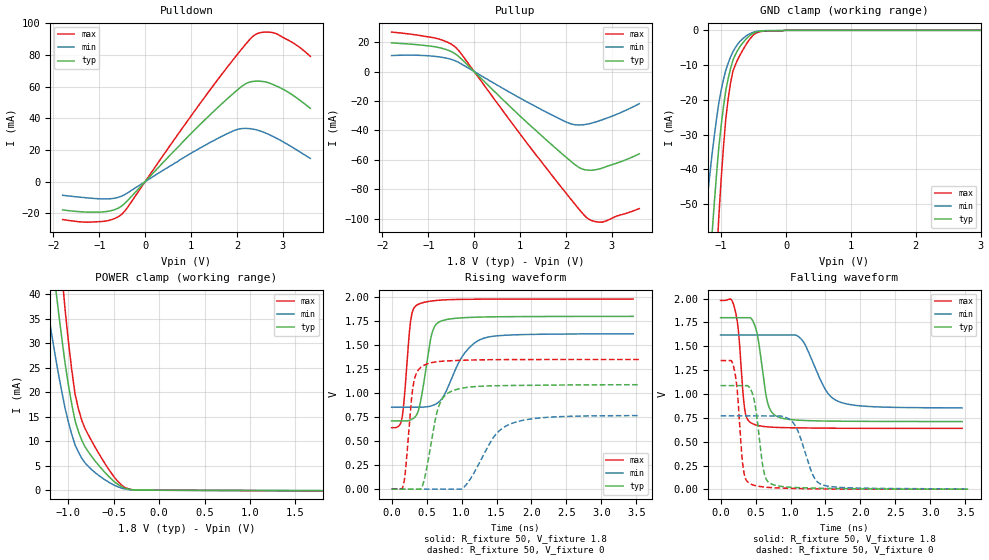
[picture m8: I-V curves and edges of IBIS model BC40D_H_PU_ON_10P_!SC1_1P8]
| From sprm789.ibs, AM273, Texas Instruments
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|   Model Cell BC40D_H_PU_ON_10P_!SC1_1P8
|BC40D_H_PU_ON_10P_!SC1_1P8
[Model]   BC40D_H_PU_ON_10P_!SC1_1P8
Model_type   I/O
Polarity   Non-Inverting
Enable   Active-Low
Vinl =  0.63
Vinh =  1.17
Cref =  15pF
Rref =  100.0000M
Vref =  0V
Vmeas =  0.9
C_comp   2.389419p   2.292106p   2.408415p
|[Input load] weak_pu_on
|[Output drive] fast
|[supplytol] 10
|[temp] ind
[Model Spec]
Vinl   0.63   0.567   0.693
Vinh   1.17   1.053   1.287
[Temperature Range]   25   125   -40
[Voltage Range]   1.8   1.62   1.98
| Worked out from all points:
|   slope of the pulldown table from 0 to 0.27 V, typ, clamps not added: 32.2 ohm
|   slope of the pullup table from 0 to 0.27 V, typ, clamps not added: 32.5 ohm
|   GND clamp passes 1 mA (typ) near -0.52 V on its own axis
|   POWER clamp passes 1 mA (typ) near -0.44 V on its own axis
|   rising waveform, R_fixture 50, V_fixture 1.8: 20-80 % time 145ps typ, 330ps min, 88.9ps max; typ from 0.711 V to 1.8 V
|   rising waveform, R_fixture 50, V_fixture 0: 20-80 % time 176ps typ, 382ps min, 100ps max; typ from 0 V to 1.09 V
|   falling waveform, R_fixture 50, V_fixture 1.8: 20-80 % time 130ps typ, 293ps min, 86ps max; typ from 1.8 V to 0.711 V
|   falling waveform, R_fixture 50, V_fixture 0: 20-80 % time 113ps typ, 213ps min, 82.9ps max; typ from 1.09 V to 0.002 V
| Nom Voltages:
|   VDD=1.1001, VDDS=1.8, VDDS18=1.8, ESD_BIASFET=0, VSS=0, VSSS=0
| Min Voltages:
|   VDD=0.99, VDDS=1.62, VDDS18=1.62, ESD_BIASFET=0, VSS=0, VSSS=0
| Max Voltages:
|   VDD=1.21, VDDS=1.98, VDDS18=1.98, ESD_BIASFET=0, VSS=0, VSSS=0
[POWER_clamp]
|   voltage   I(typ)   I(min)   I(max)
-1.8V     158.8mA    112.5mA    219.8mA
-1.255V   59.97mA    40.01mA    84.9mA
-1.145V   41.92mA    27.42mA    59.75mA
-1.109V   36.32mA    23.63mA    51.82mA
-1.073V   30.96mA    20.05mA    44.15mA
-1.036V   25.83mA    16.67mA    36.75mA
-963.6mV  17.54mA    11.39mA    24.55mA
-890.9mV  12.01mA    7.801mA    16.66mA
-818.2mV  8.875mA    5.6mA      12.63mA
-563.6mV  2.954mA    1.727mA    4.458mA
-272.7mV  55.97uA    39.41uA    57.82uA
1.8V      -99.94uA   -59.68uA   -146.8uA
[Pulldown]
|   voltage   I(typ)   I(min)   I(max)
-1.8V     -17.92mA   -8.674mA   -24.03mA
-927.3mV  -19.22mA   -10.99mA   -25.21mA
-654.5mV  -17.65mA   -10.46mA   -23.22mA
-490.9mV  -14.97mA   -8.904mA   -20.12mA
818.2mV   25.05mA    14.78mA    34.16mA
1.691V    49.7mA     28.87mA    68.59mA
2.127V    60.63mA    33.53mA    84.59mA
2.4V      63.43mA    32.84mA    92.9mA
2.618V    62.99mA    30.74mA    94.47mA
2.836V    60.69mA    27.76mA    93.76mA
3.273V    53.49mA    20.53mA    86.73mA
3.6V      46.26mA    14.64mA    79.11mA
[Pullup]
|   voltage   I(typ)   I(min)   I(max)
-1.8V     19.47mA    10.86mA    26.81mA
-818.2mV  16.61mA    10.18mA    22.5mA
-545.5mV  14.21mA    8.665mA    19.39mA
-381.8mV  11.35mA    6.855mA    15.77mA
1.036V    -31.31mA   -18.66mA   -43.94mA
1.909V    -55.72mA   -32.86mA   -78.99mA
2.182V    -62.87mA   -36.1mA    -89.59mA
2.345V    -66.12mA   -36.26mA   -95.76mA
2.455V    -66.95mA   -35.82mA   -99.33mA
2.618V    -66.9mA    -34.58mA   -101.8mA
2.782V    -65.73mA   -32.89mA   -102.4mA
3.6V      -55.92mA   -21.86mA   -93.15mA
[GND_clamp]
|   voltage   I(typ)   I(min)   I(max)
-1.8V     -270.2mA   -170.2mA   -430.1mA
-1.255V   -91.68mA   -55.92mA   -148.5mA
-1.145V   -59.94mA   -36.46mA   -97.15mA
-1.109V   -50.51mA   -30.84mA   -81.62mA
-1.073V   -41.77mA   -25.67mA   -67.14mA
-1.036V   -33.71mA   -20.94mA   -53.69mA
-927.3mV  -17.15mA   -11.38mA   -25.2mA
-854.5mV  -10.96mA   -7.657mA   -15.09mA
-781.8mV  -7.031mA   -4.995mA   -9.958mA
-563.6mV  -1.569mA   -1.036mA   -2.651mA
-18.18mV  0A         0A         0A
3.6V      0A         0A         0A
[Ramp]
| variable   typ   min   max
dV/dt_f 0.66463363/0.13264571n 0.47012824/0.29953481n 0.81358705/87.601634p
dV/dt_r 0.66384837/0.1782439n 0.48059819/0.39802224n 0.81799537/0.10135541n
R_load = 50
[Rising Waveform]
R_fixture = 50
V_fixture = 1.8
V_fixture_min = 1.62
V_fixture_max = 1.98
|   time   V(typ)   V(min)   V(max)
0s        710.5mV    852.8mV    640.5mV
143.5ps   710.5mV    852.8mV    721.7mV
179.2ps   710.5mV    852.8mV    931.5mV
273.6ps   722.6mV    852.8mV    1.76V
373.4ps   799.3mV    852.8mV    1.923V
571.2ps   1.607V     868.2mV    1.96V
697.6ps   1.748V     923.5mV    1.969V
1.016ns   1.785V     1.389V     1.977V
1.312ns   1.793V     1.571V     1.979V
3.453ns   1.8V       1.618V     1.98V
[Rising Waveform]
R_fixture = 50
V_fixture = 0
V_fixture_min = 0
V_fixture_max = 0
|   time   V(typ)   V(min)   V(max)
0s        0V         0V         3.403mV
168.2ps   0V         0V         41.85mV
312.5ps   0V         0V         1.097V
465.8ps   95.89mV    0V         1.292V
662.5ps   837mV      0V         1.328V
859.1ps   1.021V     0V         1.338V
1.051ns   1.057V     33.52mV    1.343V
1.47ns    1.077V     552.6mV    1.349V
1.714ns   1.08V      683.4mV    1.35V
3.542ns   1.088V     766.1mV    1.351V
[Falling Waveform]
R_fixture = 50
V_fixture = 1.8
V_fixture_min = 1.62
V_fixture_max = 1.98
|   time   V(typ)   V(min)   V(max)
0s        1.8V       1.619V     1.981V
202.5ps   1.8V       1.619V     1.896V
255.7ps   1.8V       1.619V     1.659V
347ps     1.8V       1.619V     831.8mV
449.6ps   1.781V     1.619V     691.7mV
673.3ps   907.3mV    1.619V     655.6mV
807.1ps   765.1mV    1.619V     649.8mV
1.149ns   724.1mV    1.58V      645mV
1.693ns   715.1mV    919.7mV    641.1mV
3.453ns   711.3mV    854.8mV    639.8mV
[Falling Waveform]
R_fixture = 50
V_fixture = 0
V_fixture_min = 0
V_fixture_max = 0
|   time   V(typ)   V(min)   V(max)
0s        1.089V     770.9mV    1.351V
189.1ps   1.089V     770.9mV    1.278V
238.1ps   1.089V     770.9mV    1.041V
324.3ps   1.089V     770.9mV    219.8mV
426.3ps   1.055V     770.9mV    58.32mV
620.7ps   180.8mV    770.9mV    25.08mV
727.2ps   56.45mV    770.9mV    18.62mV
1.045ns   20.85mV    692.9mV    9.8mV
1.455ns   11.72mV    48.64mV    4.319mV
3.542ns   2.494mV    4.994mV    2.572mV
